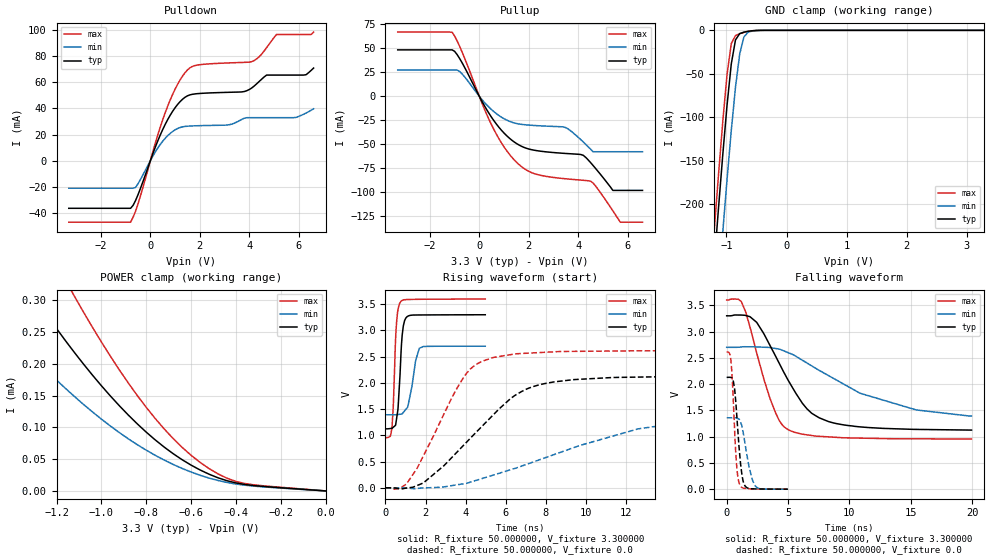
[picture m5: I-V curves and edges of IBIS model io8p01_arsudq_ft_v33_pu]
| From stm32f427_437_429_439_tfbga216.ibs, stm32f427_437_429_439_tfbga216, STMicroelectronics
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|   Model io8p01_arsudq_ft_v33_pu
[Model]  io8p01_arsudq_ft_v33_pu
Model_type I/O
Polarity   Non-Inverting
Enable   Active-Low
Vinl =   0.990000V
Vinh =   2.310000V
Vmeas =  1.650000V
Cref =   50.000000pF
Rref =   100.000000M
Vref =   0.0V
C_comp   2.292100pF   2.219400pF   2.369900pF
[Temperature Range]   25.000000   0.125000k   -40.000000
[Pullup Reference]   3.300000V   2.700000V   3.600000V
[Pulldown Reference]   0.0V   0.0V   0.0V
[POWER Clamp Reference]   3.300000V   2.700000V   3.600000V
[GND Clamp Reference]   0.0V   0.0V   0.0V
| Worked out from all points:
|   slope of the pulldown table from 0 to 0.495 V, typ, clamps not added: 20.9 ohm
|   slope of the pullup table from 0 to 0.495 V, typ, clamps not added: 22.6 ohm
|   GND clamp passes 1 mA (typ) near -0.62 V on its own axis
|   rising waveform, R_fixture 50.000000, V_fixture 3.300000: 20-80 % time 190ps typ, 344ps min, 161ps max; typ from 1.12 V to 3.3 V
|   rising waveform, R_fixture 50.000000, V_fixture 0.0: 20-80 % time 3.32ns typ, 6.65ns min, 2.1ns max; typ from 0.001 V to 2.13 V
|   falling waveform, R_fixture 50.000000, V_fixture 3.300000: 20-80 % time 3.19ns typ, 7.06ns min, 2.02ns max; typ from 3.3 V to 1.12 V
|   falling waveform, R_fixture 50.000000, V_fixture 0.0: 20-80 % time 435ps typ, 651ps min, 337ps max; typ from 2.13 V to 0.001 V
[Pulldown]
|Voltage   I(typ)   I(min)   I(max)
-3.3V     -36.46mA   -21.09mA   -47.09mA
-800mV    -36.46mA   -21.09mA   -47.09mA
-600mV    -30.5mA    -20.55mA   -38.69mA
700mV     31.4mA     19.11mA    41.71mA
1.2V      45.15mA    25.37mA    61.75mA
1.6V      50.35mA    26.5mA     71.06mA
3.1V      52.28mA    27.26mA    74.76mA
4.1V      55.64mA    32.89mA    75.8mA
4.7V      65.5mA     32.89mA    86.49mA
5.1V      65.5mA     32.89mA    96.54mA
6.3V      65.83mA    36.48mA    96.54mA
6.6V      70.88mA    39.69mA    98.4mA
[Pullup]
|Voltage   I(typ)   I(min)   I(max)
-3.3V     48.39mA    27.38mA    66.91mA
-1.1V     48.39mA    27.38mA    66.69mA
-700mV    35.09mA    23.45mA    46.29mA
500mV     -22.06mA   -14mA      -30.03mA
1.5V      -49.1mA    -28.3mA    -68.56mA
2.2V      -56.04mA   -30.32mA   -80.35mA
3.5V      -59.52mA   -32.65mA   -85.91mA
4.2V      -61.43mA   -47.47mA   -87.45mA
4.5V      -69.06mA   -55.01mA   -88.37mA
5.4V      -98mA      -57.7mA    -119.2mA
5.7V      -98mA      -57.7mA    -131.1mA
6.6V      -98mA      -57.7mA    -131.1mA
[GND_clamp]
|Voltage   I(typ)   I(min)   I(max)
-3.3V     -2.314A    -2.394A    -2.288A
-1.2V     -265.5mA   -356.1mA   -227.2mA
-1.13V    -202.6mA   -292.9mA   -164.1mA
-1.06V    -142.2mA   -231.2mA   -104.1mA
-990mV    -85.98mA   -171.6mA   -50.72mA
-920mV    -38.8mA    -115.5mA   -15.28mA
-850mV    -11.08mA   -65.6mA    -6.001mA
-780mV    -3.782mA   -27.42mA   -3.876mA
-710mV    -2.086mA   -7.69mA    -2.381mA
-640mV    -1.147mA   -2.118mA   -1.22mA
-570mV    -523.9uA   -798.4uA   -476.8uA
3.28V     0A         0A         0A
[POWER_clamp]
|Voltage   I(typ)   I(min)   I(max)
-3.28V    785.2uA    403.2uA    1.133mA
-1.56V    448.2uA    307.3uA    613.5uA
-1.32V    315.9uA    216.2uA    438.6uA
-1.28V    295.2uA    201.9uA    411uA
-1.12V    217.7uA    148.5uA    306.1uA
-960mV    149.4uA    102.1uA    211.9uA
-800mV    92.4uA     64.03uA    131.4uA
-680mV    58.5uA     41.61uA    82.28uA
-560mV    32.91uA    24.62uA    44.81uA
-440mV    16uA       13.27uA    19.94uA
-360mV    10.09uA    8.954uA    11.61uA
0V        0A         0A         0A
[Ramp]
| variable   typ   min   max
dV/dt_r  1.27849/3.32584n   0.80097/6.67459n   1.56676/2.09634n
dV/dt_f  1.30182/3.19186n   0.74298/7.04672n   1.58711/2.01788n
R_load = 50.000000
[Rising Waveform]
R_fixture= 50.000000
V_fixture= 3.300000
V_fixture_min= 2.700000
V_fixture_max= 3.600000
|time   V(typ)   V(min)   V(max)
0s        1.125V     1.393V     955.5mV
320.3ps   1.134V     1.393V     1.123V
550.6ps   1.31V      1.395V     3.136V
630.6ps   1.535V     1.399V     3.406V
750.8ps   2.362V     1.405V     3.544V
830.8ps   2.896V     1.411V     3.572V
961ps     3.194V     1.471V     3.587V
1.111ns   3.271V     1.54V      3.59V
1.692ns   3.296V     2.661V     3.595V
4.985ns   3.3V       2.7V       3.599V
[Rising Waveform]
R_fixture= 50.000000
V_fixture= 0.0
V_fixture_min= 0.0
V_fixture_max= 0.0
|time   V(typ)   V(min)   V(max)
0s        1.283mV    1.128mV    1.883mV
480.5ps   -4.042mV   1.255mV    -25.28mV
1.081ns   -2.69mV    -4.199mV   92.02mV
1.922ns   103mV      -218.1uV   631.1mV
3.844ns   788.8mV    74.01mV    2.07V
4.845ns   1.182V     179.8mV    2.416V
6.486ns   1.767V     372.9mV    2.554V
8.408ns   2.019V     632mV      2.593V
12.61ns   2.111V     1.123V     2.612V
19.94ns   2.129V     1.36V      2.612V
[Falling Waveform]
R_fixture= 50.000000
V_fixture= 3.300000
V_fixture_min= 2.700000
V_fixture_max= 3.600000
|time   V(typ)   V(min)   V(max)
0s        3.3V       2.7V       3.599V
1.201ns   3.314V     2.708V     3.567V
2.442ns   3.176V     2.707V     2.596V
3.524ns   2.737V     2.695V     1.729V
4.284ns   2.394V     2.667V     1.306V
5.005ns   2.074V     2.599V     1.134V
6.527ns   1.533V     2.404V     1.035V
8.689ns   1.262V     2.111V     990.6mV
15.42ns   1.138V     1.51V      958.8mV
19.94ns   1.125V     1.393V     955.5mV
[Falling Waveform]
R_fixture= 50.000000
V_fixture= 0.0
V_fixture_min= 0.0
V_fixture_max= 0.0
|time   V(typ)   V(min)   V(max)
0s        2.129V     1.36V      2.612V
340.3ps   2.126V     1.359V     2.458V
550.6ps   2.045V     1.359V     1.622V
810.8ps   1.438V     1.354V     456.9mV
1.071ns   636.8mV    1.307V     84.8mV
1.251ns   260.8mV    1.185V     31.36mV
1.431ns   89.72mV    963mV      16.88mV
1.822ns   14.53mV    426.4mV    8.53mV
2.332ns   5.851mV    61.16mV    5.107mV
4.985ns   1.283mV    1.128mV    1.883mV
